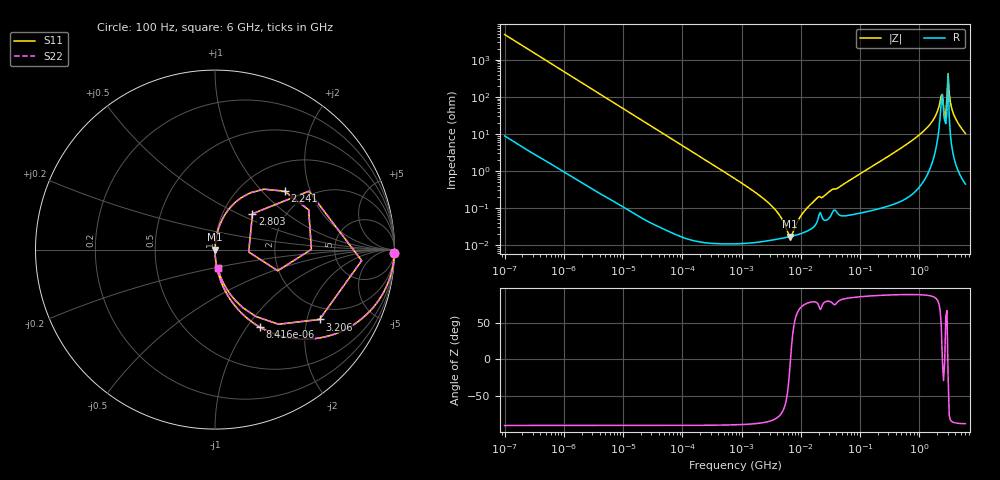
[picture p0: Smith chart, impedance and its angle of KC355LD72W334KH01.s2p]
!Murata Part Number: KC355LD72W334KH01
!These Parameters are Measured in Series Mode Connection
!Data Generated on Mar 13, 2026
!  o--ll--o
!Port1  Port2
!  o------o
!Operation Temp=25[degC], DC Bias Voltage=0[V]
!Freq. Start=100[Hz] Stop=6[GHz] 401[Steps]
# Hz S RI R 50
!Freq.(Hz) S11(Real) S11(Imag) S21(Real) S21(Imag) S12(Real) S12(Imag) S22(Real) S22(Imag)
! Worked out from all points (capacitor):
!   401 points, 100 Hz to 6 GHz, reference 50 ohm
!   read as one part in series: C = 330 nF near 109 Hz
!   lowest |Z| = 17.1 mohm at 6.644 MHz (marker M1)
!   series resonance near 6.702 MHz, so ESL is about 1.7 nH
!   S11 on the Smith chart (normalised r, x): 100 Hz: 1, -96; 8.416 kHz: 1.00, -1.15; 2.241 GHz: 1.55, +1.36; 2.803 GHz: 1.38, +0.60; 3.206 GHz: 1.56, -2.39; 6 GHz: 1.01, -0.20
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100  0.9995 -0.0207  0.000468 0.0207  0.000468 0.0207  0.9995 -0.0207
548  0.9871 -0.112  0.0129 0.112  0.0129 0.112  0.9871 -0.112
2008  0.8525 -0.3536  0.1475 0.3536  0.1475 0.3536  0.8525 -0.3536
4299  0.559 -0.4955  0.441 0.4955  0.441 0.4955  0.559 -0.4955
8416  0.2495 -0.4316  0.7505 0.4316  0.7505 0.4316  0.2495 -0.4316
40335  0.0146 -0.1186  0.9854 0.1186  0.9854 0.1186  0.0146 -0.1186
774597  0.000147 -0.00618  0.9999 0.00618  0.9999 0.00618  0.000147 -0.00618
3245845  0.000138 -0.00113  0.9999 0.00113  0.9999 0.00113  0.000138 -0.00113
4440638  0.00015 -0.000602  0.9998 0.000602  0.9998 0.000602  0.00015 -0.000602
6644369  0.000171 -1.21e-05  0.9998 1.21e-05  0.9998 1.21e-05  0.000171 -1.21e-05
1.039699e7  0.00021 0.00064  0.9998 -0.00064  0.9998 -0.00064  0.00021 0.00064
1.555665e7  0.000289 0.00135  0.9997 -0.00135  0.9997 -0.00135  0.000289 0.00135
3.124326e8  0.00183 0.0259  0.9982 -0.0259  0.9982 -0.0259  0.00183 0.0259
1.565993e9  0.0478 0.182  0.9522 -0.182  0.9522 -0.182  0.0478 0.182
1.95892e9  0.1449 0.2884  0.8551 -0.2884  0.8551 -0.2884  0.1449 0.2884
2.240541e9  0.3887 0.3251  0.6113 -0.3251  0.6113 -0.3251  0.3887 0.3251
2.450438e9  0.5372 0.00144  0.4628 -0.00144  0.4628 -0.00144  0.5372 0.00144
2.802721e9  0.2089 0.1998  0.7911 -0.1998  0.7911 -0.1998  0.2089 0.1998
3.205649e9  0.5826 -0.3891  0.4174 0.3891  0.4174 0.3891  0.5826 -0.3891
3.505958e9  0.2273 -0.3724  0.7727 0.3724  0.7727 0.3724  0.2273 -0.3724
4.009986e9  0.0856 -0.2496  0.9144 0.2496  0.9144 0.2496  0.0856 -0.2496
6e9  0.0146 -0.1003  0.9854 0.1003  0.9854 0.1003  0.0146 -0.1003
